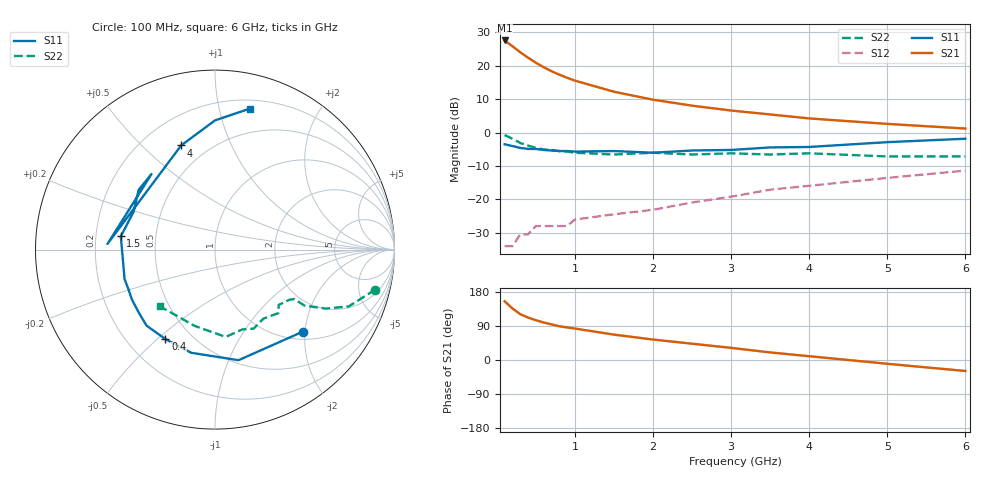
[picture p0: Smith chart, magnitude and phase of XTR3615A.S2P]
! HXTR-3615 Common Emitter
! Vce=10V  Ic=10mA
# ghz s ma r 50
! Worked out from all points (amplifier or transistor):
!   18 points, 100 MHz to 6 GHz, reference 50 ohm
!   highest |S21| = 27.6 dB at 100 MHz (marker M1)
!   |S21| within 3 dB of that: start of sweep to 270.9 MHz
!   unconditionally stable (mu >= 1): 1.456 GHz to 2.984 GHz
!   at 400 MHz: K = 0.45, MSG = 26.4 dB, |S12| = -30.5 dB
!   at 1 GHz: K = 0.83, MSG = 20.8 dB, |S12| = -26.0 dB
!   at 6 GHz: K = 0.43, MSG = 6.3 dB, |S12| = -11.4 dB
!   lowest NFmin = 1.40 dB at 1 GHz
!   S11 on the Smith chart (normalised r, x): 100 MHz: 1.18, -1.95; 400 MHz: 0.36, -0.53; 1.5 GHz: 0.31, +0.06; 4 GHz: 0.36, +0.66; 6 GHz: 0.27, +1.24
0.1  0.67 -43.0  23.92 155.0  0.02 66.0  0.92 -14.0
0.2  0.63 -78.0  19.63 136.0  0.02 70.0  0.81 -23.0
0.3  0.59 -103.0  15.94 121.0  0.03 53.0  0.7 -28.0
0.4  0.57 -119.0  13.22 112.0  0.03 52.0  0.64 -30.0
0.5  0.57 -132.0  11.11 105.0  0.04 46.0  0.59 -32.0
0.6  0.55 -141.0  9.52 99.0  0.04 49.0  0.56 -32.0
0.7  0.54 -149.0  8.3 94.0  0.04 50.0  0.55 -32.0
0.8  0.53 -156.0  7.37 89.0  0.04 49.0  0.53 -32.0
0.9  0.53 -162.0  6.61 86.0  0.04 51.0  0.52 -32.0
1  0.52 -168.0  6 83.0  0.05 50.0  0.5 -34.0
1.5  0.53 172.0  4.09 67.0  0.06 55.0  0.47 -41.0
2  0.5 155.0  3.11 54.0  0.07 58.0  0.5 -45.0
2.5  0.54 142.0  2.53 43.0  0.09 59.0  0.47 -55.0
3  0.55 130.0  2.14 32.0  0.11 58.0  0.49 -64.0
3.5  0.6 177.0  1.87 20.0  0.14 56.0  0.47 -71.0
4  0.61 108.0  1.63 10.0  0.16 52.0  0.49 -83.0
5  0.72 90.0  1.35 -10.0  0.21 43.0  0.44 -105.0
6  0.81 76.0  1.15 -29.0  0.27 32.0  0.44 -134.0
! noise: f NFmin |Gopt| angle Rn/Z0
1  1.4  0.2  135  0.308
2  2  0.39  -177  0.094
4  3.5  0.54  -116  0.362
